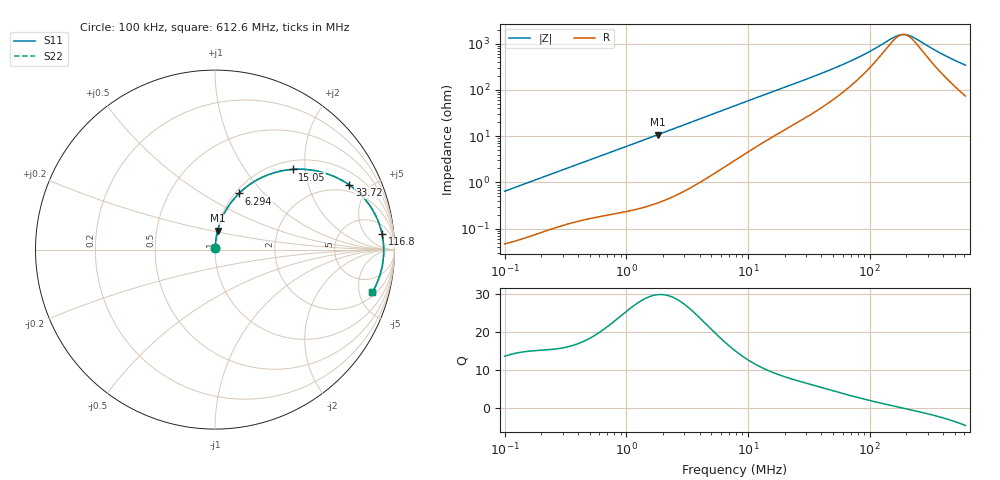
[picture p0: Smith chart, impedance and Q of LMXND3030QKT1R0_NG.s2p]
! LMXND3030QKT1R0_NG  S-PARAMETER MODEL  ( General Type )
! Model Generated by TAIYO YUDEN Corporation (http://www.ty-top.com)
! Version 1.0
! TAIYO YUDEN Control No. 191023NI43SB-FBB
! Copyright(c) 2019 TAIYO YUDEN CO.,LTD. All Rights Reserved.
! Product Description (link to TY-COMPAS)
! https://ds.yuden.co.jp/TYCOMPAS/or/detail?pn=LMXND3030QKT1R0NNG&u=M
! Products Name : Inductors
! Characteristics :
!  Inductance : 1.0 uH , SRF(min) : 100 MHz , DC Resistance(max) : 0.036 Ohm
!  Rated Current : Saturation :2100 mA , Temp Rise : 2100 mA
!  Case Size : 3.0 x 3.0 / 0.118 x 0.118 [mm/inch] , Thickness : 1.5 / 0.059 [mm/inch]
!  (Conditions: Temperature = 25 degC , DC Bias Current/Voltage = 0A / 0V)
! External Node Assignments :
!  1  o---GGG---o  2
! GND o---------o GND
! Frequency Range : 0.1MHz  -  612.621916MHz  [ 402 STEP ]
# MHz S RI R 50
! Freq[MHz].  S11 Real  S11 Imag  S21 Real  S21 Imag  S12 Real  S12 Imag  S22 Real  S22 Imag
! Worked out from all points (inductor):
!   401 points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, 100 kHz to 612.6 MHz, reference 50 ohm
!   read as one part in series: L = 1.01 uH near 104.5 kHz
!   highest Q = 29.9 at 1.817 MHz (marker M1), where L = 942 nH
!   self-resonance near 189.6 MHz
!   S11 on the Smith chart (normalised r, x): 100 kHz: 1.00, +0.01; 6.294 MHz: 1.04, +0.74; 15.05 MHz: 1.18, +1.71; 33.72 MHz: 1.61, +3.74; 116.8 MHz: 10, +14; 612.6 MHz: 2.46, -6.66
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0.1  0.000509 0.0064  0.9995 -0.0064  0.9995 -0.0064  0.000509 0.0064
0.430878  0.00219 0.0261  0.9978 -0.0261  0.9978 -0.0261  0.00219 0.0261
0.965317  0.00556 0.057  0.9944 -0.057  0.9944 -0.057  0.00556 0.057
1.816526  0.0149 0.1055  0.9851 -0.1055  0.9851 -0.1055  0.0149 0.1055
1.856562  0.0155 0.1077  0.9845 -0.1077  0.9845 -0.1077  0.0155 0.1077
3.729794  0.0536 0.206  0.9464 -0.206  0.9464 -0.206  0.0536 0.206
6.293851  0.1331 0.3126  0.8669 -0.3126  0.8669 -0.3126  0.1331 0.3126
7.827017  0.1881 0.3591  0.8119 -0.3591  0.8119 -0.3591  0.1881 0.3591
11.09389  0.3061 0.4206  0.6939 -0.4206  0.6939 -0.4206  0.3061 0.4206
15.05344  0.4322 0.4467  0.5678 -0.4467  0.5678 -0.4467  0.4322 0.4467
21.80677  0.5911 0.4323  0.4089 -0.4323  0.4089 -0.4323  0.5911 0.4323
33.72493  0.749 0.3596  0.251 -0.3596  0.251 -0.3596  0.749 0.3596
46.77036  0.8322 0.2844  0.1678 -0.2844  0.1678 -0.2844  0.8322 0.2844
66.29159  0.8885 0.2027  0.1115 -0.2027  0.1115 -0.2027  0.8885 0.2027
89.95186  0.917 0.1369  0.083 -0.1369  0.083 -0.1369  0.917 0.1369
116.8493  0.9309 0.0859  0.0691 -0.0859  0.0691 -0.0859  0.9309 0.0859
145.3134  0.9372 0.0463  0.0628 -0.0463  0.0628 -0.0463  0.9372 0.0463
176.8144  0.9398 0.012  0.0602 -0.012  0.0602 -0.012  0.9398 0.012
192.9254  0.9401 -0.00306  0.0599 0.00306  0.0599 0.00306  0.9401 -0.00306
210.5045  0.9399 -0.0182  0.0601 0.0182  0.0601 0.0182  0.9399 -0.0182
396.1256  0.9204 -0.1367  0.0796 0.1367  0.0796 0.1367  0.9204 -0.1367
612.6219  0.8772 -0.2363  0.1228 0.2363  0.1228 0.2363  0.8772 -0.2363
